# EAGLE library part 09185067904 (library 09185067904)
Connectors, Male connector, Wave soldering termination, Rated current: 1 A, Straight Source: Datasheet
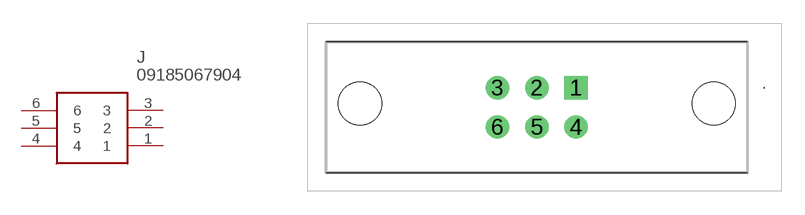
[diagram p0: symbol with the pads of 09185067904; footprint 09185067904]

Designator prefix J

## 09185067904 (Description: Connectors, Male connector, Wave soldering termination, Rated current: 1 A, Straight; Height: 25.75mm; Manufacturer_Name: HARTING; Manufacturer_Part_Number: 09185067904; Mouser_Part_Number: 617-09-18-506-7904; Mouser_Price-Stock: https://www.mouser.com/Search/Refine.aspx?Keyword=617-09-18-506-7904)  [09185067904]
1  1
2  2
3  3
4  4
5  5
6  6

## Footprint 09185067904 (pad centres in mm)
09185067904
drill 1 pad 1.5 square: 1 0,0
drill 1 pad 1.5: 2 -2.54,0; 3 -5.08,0; 4 0,-2.54; 5 -2.54,-2.54; 6 -5.08,-2.54
hole 2.8 at -13.97,-1.02
hole 2.8 at 8.89,-1.02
